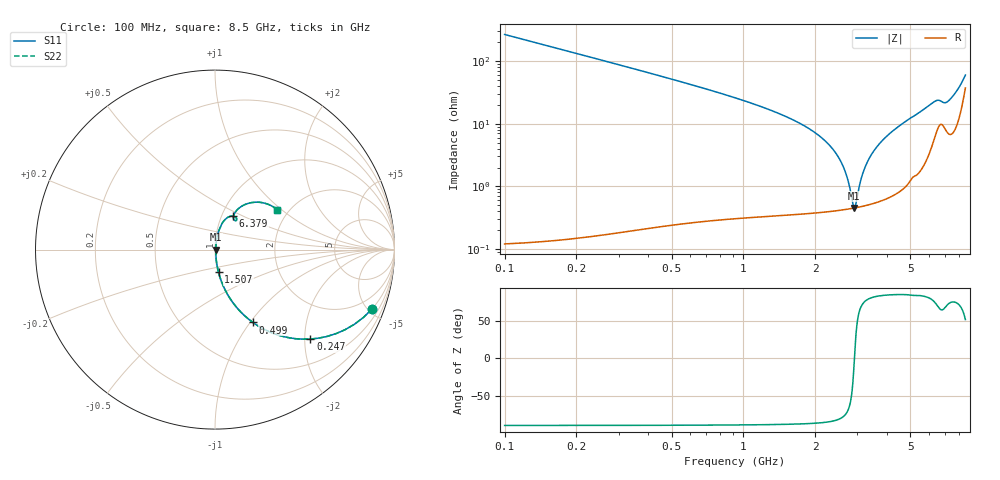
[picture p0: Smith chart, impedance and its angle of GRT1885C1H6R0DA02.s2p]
!Murata Part Number: GRT1885C1H6R0DA02
!These Parameters are Measured in Series Mode Connection
!Data Generated on Jun 19, 2026
!  o--ll--o
!Port1  Port2
!  o------o
!Operation Temp=25[degC], DC Bias Voltage=0[V]
!Freq. Start=100[MHz] Stop=9[GHz] 401[Steps]
# Hz S RI R 50
!Freq.(Hz) S11(Real) S11(Imag) S21(Real) S21(Imag) S12(Real) S12(Imag) S22(Real) S22(Imag)
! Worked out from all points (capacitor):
!   401 points, 100 MHz to 8.5 GHz, reference 50 ohm
!   read as one part in series: C = 6 pF near 142 MHz
!   lowest |Z| = 453 mohm at 2.914 GHz (marker M1)
!   series resonance near 2.916 GHz, so ESL is about 500 pH
!   S11 on the Smith chart (normalised r, x): 100 MHz: 1.00, -5.30; 247 MHz: 1.00, -2.13; 499 MHz: 1.00, -1.03; 1.507 GHz: 1.01, -0.26; 6.379 GHz: 1.13, +0.44; 8.5 GHz: 1.74, +0.93
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1e8  0.8752 -0.3303  0.1248 0.3303  0.1248 0.3303  0.8752 -0.3303
2.47e8  0.5317 -0.4982  0.4683 0.4982  0.4683 0.4982  0.5317 -0.4982
3.73e8  0.3286 -0.4682  0.6714 0.4682  0.6714 0.4682  0.3286 -0.4682
4.99e8  0.2111 -0.4057  0.7889 0.4057  0.7889 0.4057  0.2111 -0.4057
8.56e8  0.0766 -0.2608  0.9234 0.2608  0.9234 0.2608  0.0766 -0.2608
1.507e9  0.0199 -0.1269  0.9801 0.1269  0.9801 0.1269  0.0199 -0.1269
2.095e9  0.00764 -0.0616  0.9924 0.0616  0.9924 0.0616  0.00764 -0.0616
2.452e9  0.00512 -0.0322  0.9949 0.0322  0.9949 0.0322  0.00512 -0.0322
2.683e9  0.00451 -0.0155  0.9955 0.0155  0.9955 0.0155  0.00451 -0.0155
2.767e9  0.00445 -0.00982  0.9956 0.00982  0.9956 0.00982  0.00445 -0.00982
2.872e9  0.00447 -0.00287  0.9955 0.00287  0.9955 0.00287  0.00447 -0.00287
2.914e9  0.0045 -0.000146  0.9955 0.000146  0.9955 0.000146  0.0045 -0.000146
2.956e9  0.00456 0.00254  0.9954 -0.00254  0.9954 -0.00254  0.00456 0.00254
3.145e9  0.00498 0.0143  0.995 -0.0143  0.995 -0.0143  0.00498 0.0143
3.376e9  0.00589 0.028  0.9941 -0.028  0.9941 -0.028  0.00589 0.028
3.754e9  0.00824 0.0494  0.9918 -0.0494  0.9918 -0.0494  0.00824 0.0494
4.3e9  0.0136 0.0791  0.9864 -0.0791  0.9864 -0.0791  0.0136 0.0791
5.707e9  0.0477 0.158  0.9523 -0.158  0.9523 -0.158  0.0477 0.158
6.379e9  0.1011 0.1863  0.8989 -0.1863  0.8989 -0.1863  0.1011 0.1863
7.114e9  0.1027 0.1746  0.8973 -0.1746  0.8973 -0.1746  0.1027 0.1746
7.828e9  0.1592 0.2474  0.8408 -0.2474  0.8408 -0.2474  0.1592 0.2474
8.5e9  0.3467 0.2227  0.6533 -0.2227  0.6533 -0.2227  0.3467 0.2227
